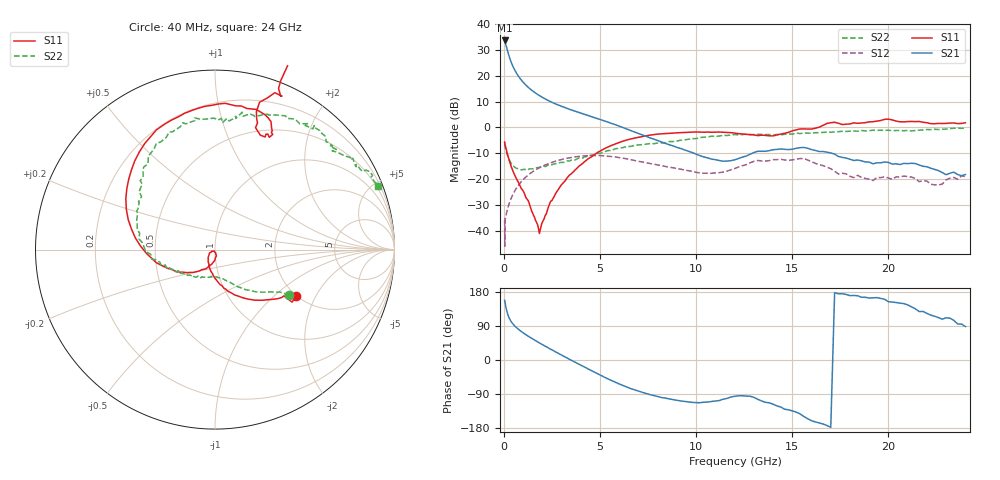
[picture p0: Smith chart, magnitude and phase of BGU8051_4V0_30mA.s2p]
! BGU8051_4V0_30mA
! Date/time Tue Jun 16 10:58:09 2015
! VAR V_out= 4.0000
! VAR I_out= 30.0000
! VAR V_in= 3.7920
! VAR I_in= 0.3989
# MHz S MA R 50
!  Freq-MHz  S11-mag  S11-arg  S21-mag  S21-arg  S12-mag  S12-arg  S22-mag  S22-arg
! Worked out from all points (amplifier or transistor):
!   187 points, 40 MHz to 24 GHz, reference 50 ohm
!   highest |S21| = 33.6 dB at 40 MHz (marker M1)
!   |S21| within 3 dB of that: start of sweep to 154.6 MHz
!   unconditionally stable (mu >= 1): 44 MHz to 57.39 MHz; 637.8 MHz to 14.06 GHz
!   at 750 MHz: K = 1.01, MAG = 20.6 dB, |S12| = -22.4 dB
!   at 5.4 GHz: K = 1.21, MAG = 3.8 dB, |S12| = -11.1 dB
!   at 24 GHz: K = -0.33, MSG = 0.4 dB, |S12| = -19.0 dB
!   lowest NFmin = 0.30 dB at 400 MHz
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40  0.5222 -29.8  48.13 157.5  0.01592 32.1  0.4856 -31.5
50  0.5193 -34.3  46.79 155.4  0.005044 -30.5  0.4672 -32.0
60  0.4628 -33.8  45.94 152.2  0.01211 54.2  0.432 -33.2
80  0.4442 -37.9  42.87 146.8  0.01747 37.4  0.4025 -35.9
120  0.3847 -47.2  38.05 136.6  0.02021 41.9  0.3518 -42.4
140  0.3575 -52.0  35.8 132.1  0.02225 45.3  0.3324 -45.2
180  0.3116 -59.8  31.41 124.5  0.02563 48.8  0.2963 -49.9
240  0.2572 -69.5  26.2 115.4  0.03051 52.8  0.2567 -55.9
300  0.2195 -77.2  22.24 108.5  0.03557 54.8  0.2288 -60.4
360  0.1855 -84.0  19.18 103.0  0.0408 57.1  0.207 -64.0
440  0.1529 -91.5  16.14 97.2  0.04788 58.2  0.1892 -68.9
550  0.1228 -100.6  13.23 90.6  0.05772 58.6  0.1708 -73.7
750  0.08742 -112.9  9.901 81.4  0.0756 57.7  0.1585 -81.6
950  0.06275 -127.1  7.901 73.6  0.09309 55.1  0.1514 -88.3
1600  0.01807 -149.3  4.762 52.4  0.1472 43.5  0.1604 -108.5
2600  0.04491 -86.6  2.95 23.9  0.2171 22.4  0.1962 -131.3
4100  0.2016 -140.4  1.841 -16.4  0.2798 -11.0  0.2553 -154.3
8200  0.7532 111.9  0.5234 -99.0  0.1818 -76.6  0.5027 148.0
12200  0.7578 65.5  0.2502 -94.5  0.171 -71.3  0.7191 103.2
16200  0.9659 68.5  0.3581 -163.3  0.2019 -150.5  0.7914 71.0
20200  1.396 33.7  0.195 153.1  0.09914 -155.9  0.8622 44.1
24000  1.231 20.6  0.1226 88.3  0.1118 -170.2  0.9727 21.4
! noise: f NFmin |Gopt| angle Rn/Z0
400  0.298  0.204  20.62  0.0582
550  0.3118  0.1661  29.66  0.0558
950  0.3585  0.1045  69.17  0.0505
1250  0.4033  0.1027  106  0.0476
1600  0.4662  0.1274  135.1  0.0455
1900  0.5291  0.152  150.4  0.0449
2250  0.613  0.1774  163.6  0.0459
2600  0.7084  0.1988  174.7  0.0488
3300  0.9331  0.2376  194.3  0.0611
4000  1.203  0.2839  210.5  0.0833
